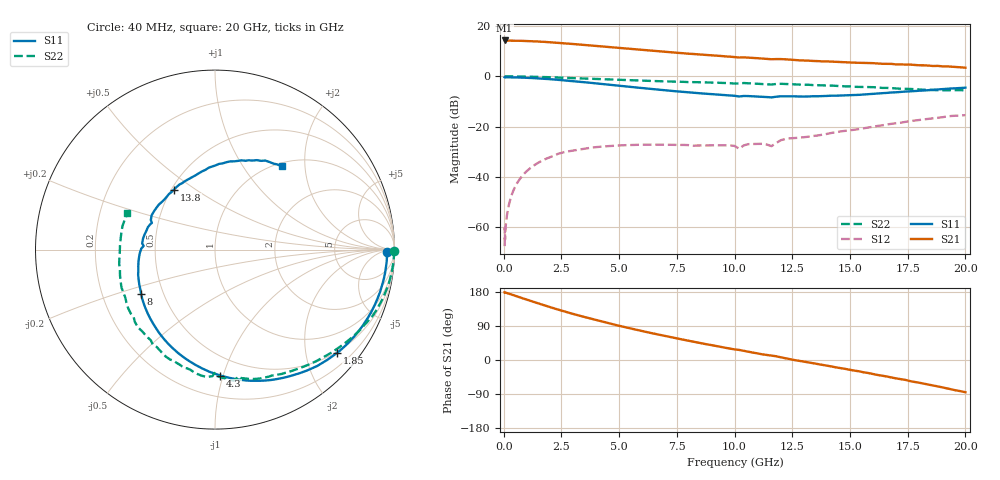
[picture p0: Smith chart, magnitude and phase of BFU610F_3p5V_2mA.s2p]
! Filename:  P:\Prog\Test\Noise\ATS_data\Testdata_Net\SplitFiles\BFU610_2W_A5_HighFreq_3.5V_2mA_D.s2p
! Date/Time: Wed 10/Aug/2011 16:56:27
! BFU610_2W_A5_HighFreq_Bias2_3.5V_1mA_10mA_R.s2p
! MDIF S-parameter v. bias file
! BFU610_2W_A5_HighFreq_3.5V_1mA_10mA
! Date/time Mon Aug 08 14:10:09 2011
! VAR V_out= 3.5010
! VAR I_out= 2.0000
! VAR V_in= 0.8642
! VAR I_in= 0.0147
! Device data file deembeded for feedlines and parallel
! Original file: \SplitFiles\BFU610_2W_A5_HighFreq_3.5V_2mA_R.s2p
! Feed-files: PR003V01_101208_Feed1.s2p, PR003V01_101208_Feed2.s2p
! Parallel-file: PR003V01_101208_Par.s2p
# MHz S MA R 50
!  Freq-MHz  S11-mag  S11-arg  S21-mag  S21-arg  S12-mag  S12-arg  S22-mag  S22-arg
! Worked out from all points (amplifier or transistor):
!   167 points, 40 MHz to 20 GHz, reference 50 ohm
!   highest |S21| = 14.3 dB at 40 MHz (marker M1)
!   |S21| within 3 dB of that: start of sweep to 5.045 GHz
!   unconditionally stable (mu >= 1): 6.934 GHz to 18.31 GHz
!   at 550 MHz: K = 0.00, MSG = 28.6 dB, |S12| = -42.9 dB
!   at 4.2 GHz: K = 0.50, MSG = 20.0 dB, |S12| = -28.0 dB
!   at 20 GHz: K = 0.87, MSG = 9.4 dB, |S12| = -15.4 dB
!   S11 on the Smith chart (normalised r, x): 40 MHz: 43, -15; 1.85 GHz: 0.47, -2.65; 4.3 GHz: 0.35, -0.98; 8 GHz: 0.37, -0.24; 13.8 GHz: 0.52, +0.41; 20 GHz: 1.07, +1.53
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40  0.9594 -0.8  5.173 178.6  0.0004209 90.0  0.9964 -0.3
50  0.9509 -1.1  5.149 178.8  0.0009805 61.5  0.9971 -0.5
60  0.9616 -1.1  5.16 177.9  0.0005734 75.6  0.9974 -0.5
100  0.9597 -2.2  5.13 177.4  0.001203 87.7  0.9972 -1.0
180  0.9589 -4.0  5.125 176.1  0.002202 90.5  0.9973 -1.8
480  0.9536 -10.7  5.108 169.9  0.006185 86.4  0.9955 -5.0
1150  0.9293 -25.4  5.021 156.3  0.01497 75.6  0.9841 -12.0
1850  0.8905 -40.4  4.82 142.5  0.02316 65.2  0.9651 -18.9
2700  0.8259 -57.7  4.526 126.9  0.03175 53.1  0.9317 -26.8
3400  0.7724 -71.1  4.252 115.0  0.03601 45.5  0.9061 -32.8
4300  0.7024 -87.5  3.929 100.7  0.04027 36.8  0.8739 -39.8
5400  0.6237 -106.6  3.549 84.6  0.04303 28.5  0.8389 -47.9
6800  0.5378 -129.8  3.125 65.8  0.04375 21.2  0.8001 -57.6
8000  0.4795 -149.2  2.82 50.9  0.04296 17.6  0.7696 -65.8
9400  0.4314 -171.1  2.545 34.5  0.04248 19.4  0.7433 -75.6
10200  0.3981 177.1  2.369 26.6  0.03638 21.7  0.7207 -79.5
12000  0.4016 151.5  2.205 7.1  0.05373 38.6  0.7111 -93.6
13400  0.4022 129.7  2.025 -8.5  0.06521 31.9  0.6708 -107.0
13800  0.4045 124.4  1.986 -12.6  0.06909 32.2  0.6609 -110.6
16800  0.4782 87.2  1.77 -46.1  0.1139 18.9  0.5837 -146.0
18400  0.5319 69.3  1.638 -65.2  0.143 5.7  0.5399 -171.3
20000  0.5957 51.0  1.49 -85.0  0.1696 -11.2  0.5294 157.1
